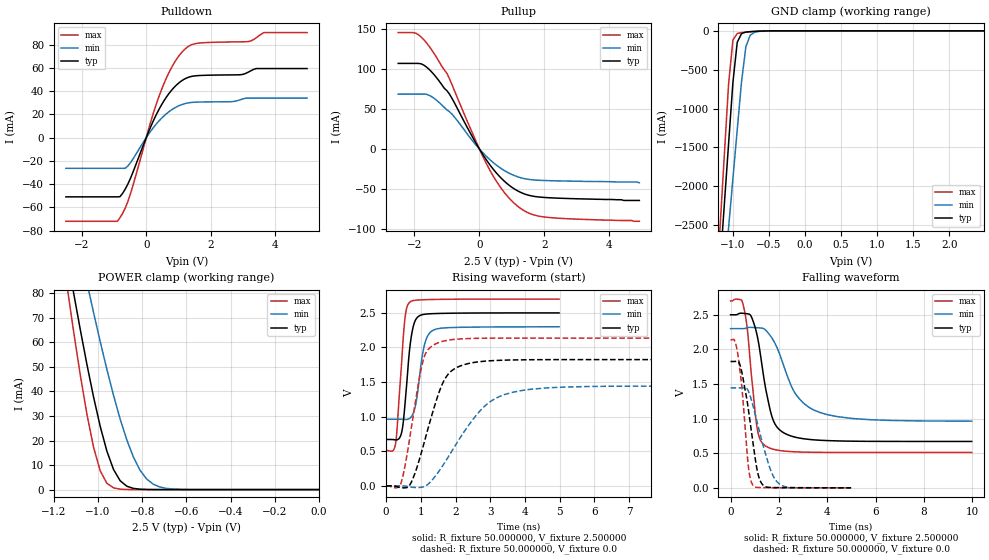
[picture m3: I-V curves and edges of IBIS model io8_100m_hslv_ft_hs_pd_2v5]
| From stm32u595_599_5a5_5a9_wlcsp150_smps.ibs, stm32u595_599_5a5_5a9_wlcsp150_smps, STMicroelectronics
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|   Model io8_100m_hslv_ft_hs_pd_2v5
[Model]  io8_100m_hslv_ft_hs_pd_2v5
Model_type I/O
Polarity   Non-Inverting
Enable   Active-Low
Vinl =   0.750000V
Vinh =   1.750000V
Vmeas =  1.250000V
Cref =   50.000000pF
Rref =   100.000000M
Vref =   0.0V
C_comp   3.340900pF   3.338500pF   3.380300pF
[Temperature Range]   25.000000   0.140000k   -40.000000
[Pullup Reference]   2.500000V   2.300000V   2.700000V
[Pulldown Reference]   0.0V   0.0V   0.0V
[POWER Clamp Reference]   2.500000V   2.300000V   2.700000V
[GND Clamp Reference]   0.0V   0.0V   0.0V
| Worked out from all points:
|   slope of the pulldown table from 0 to 0.375 V, typ, clamps not added: 16.1 ohm
|   slope of the pullup table from 0 to 0.375 V, typ, clamps not added: 16.6 ohm
|   GND clamp passes 1 mA (typ) near -0.50 V on its own axis
|   POWER clamp passes 1 mA (typ) near -0.86 V on its own axis
|   rising waveform, R_fixture 50.000000, V_fixture 2.500000: 20-80 % time 200ps typ, 230ps min, 180ps max; typ from 0.67 V to 2.5 V
|   rising waveform, R_fixture 50.000000, V_fixture 0.0: 20-80 % time 660ps typ, 1.22ns min, 424ps max; typ from 0 V to 1.82 V
|   falling waveform, R_fixture 50.000000, V_fixture 2.500000: 20-80 % time 568ps typ, 1.09ns min, 361ps max; typ from 2.5 V to 0.67 V
|   falling waveform, R_fixture 50.000000, V_fixture 0.0: 20-80 % time 467ps typ, 672ps min, 321ps max; typ from 1.82 V to 0 V
[Pulldown]
|Voltage   I(typ)   I(min)   I(max)
-2.5V     -51.01mA   -26.45mA   -72.04mA
-900mV    -51.01mA   -26.45mA   -72.04mA
-820mV    -50.89mA   -26.45mA   -69.09mA
-500mV    -35.59mA   -21.93mA   -49.09mA
140mV     9.489mA    5.639mA    13.76mA
460mV     27.5mA     16.25mA    40.22mA
860mV     43.07mA    25.18mA    63.88mA
1.26V     51.38mA    29.65mA    77.49mA
1.66V     53.45mA    30.63mA    81.42mA
3.18V     56.44mA    34.01mA    82.68mA
3.66V     59.44mA    34.01mA    90.42mA
5V        59.44mA    34.01mA    90.42mA
[Pullup]
|Voltage   I(typ)   I(min)   I(max)
-2.5V     106.7mA    68.56mA    145.2mA
-1.96V    106.7mA    68.56mA    144.4mA
-1.72V    104.8mA    68.56mA    136.6mA
-1.48V    96.52mA    65.55mA    124.2mA
-1V       72.68mA    48.88mA    94.22mA
-120mV    8.307mA    5.657mA    10.97mA
280mV     -17.4mA    -11.68mA   -23.32mA
680mV     -36.72mA   -24.56mA   -49.54mA
1.16V     -51.75mA   -34.32mA   -70.71mA
1.56V     -58mA      -38.01mA   -80.45mA
1.96V     -60.18mA   -39.11mA   -84.44mA
4.92V     -64mA      -42mA      -90mA
[GND_clamp]
|Voltage   I(typ)   I(min)   I(max)
-2.5V     -9.446A    -9.524A    -9.146A
-1.18V    -3.045A    -3.8A      -2.552A
-1.12V    -2.248A    -3.166A    -1.614A
-1.06V    -1.452A    -2.533A    -685.4mA
-1V       -665mA     -1.901A    -117.9mA
-940mV    -148mA     -1.272A    -34.34mA
-880mV    -35.14mA   -651.5mA   -22.8mA
-820mV    -16.02mA   -203.9mA   -17.08mA
-760mV    -10.47mA   -56.89mA   -12.28mA
-700mV    -7.079mA   -18.53mA   -8.16mA
-400mV    -112.4uA   -382.5uA   -53.84uA
2.48V     63.1uA     48.03uA    77.39uA
[POWER_clamp]
|Voltage   I(typ)   I(min)   I(max)
-2.49V    881mA      773.1mA    1.07A
-1.14V    95.25mA    122.7mA    82.82mA
-1.11V    79.9mA     109.7mA    64.14mA
-1.05V    50.87mA    84.26mA    30.57mA
-1.02V    37.63mA    72.04mA    17.17mA
-990mV    25.71mA    60.25mA    7.621mA
-930mV    8.217mA    38.43mA    713.9uA
-900mV    3.624mA    28.77mA    182.8uA
-840mV    490.7uA    13.24mA    11.35uA
-780mV    56.55uA    4.324mA    699nA
-660mV    716.5nA    226uA      9.775nA
0V        0A         19.49nA    0A
[Ramp]
| variable   typ   min   max
dV/dt_r  1.09464/0.65907n   0.86544/1.21762n   1.28142/0.42296n
dV/dt_f  1.09786/0.56759n   0.80138/1.08495n   1.31323/0.36111n
R_load = 50.000000
[Rising Waveform]
R_fixture= 50.000000
V_fixture= 2.500000
V_fixture_min= 2.300000
V_fixture_max= 2.700000
|time   V(typ)   V(min)   V(max)
0s        669.6mV    962.6mV    510.3mV
270.3ps   664.1mV    962.9mV    606.1mV
310.3ps   664.7mV    962.9mV    793.2mV
450.5ps   779.9mV    962.3mV    1.814V
550.6ps   1.223V     959.4mV    2.454V
680.7ps   1.991V     975.8mV    2.655V
860.9ps   2.409V     1.2V       2.683V
1.071ns   2.477V     1.964V     2.689V
1.301ns   2.487V     2.233V     2.693V
4.985ns   2.499V     2.299V     2.698V
[Rising Waveform]
R_fixture= 50.000000
V_fixture= 0.0
V_fixture_min= 0.0
V_fixture_max= 0.0
|time   V(typ)   V(min)   V(max)
0s        -146.1uV   -65.63uV   -358.7uV
400.4ps   -24.12mV   -179.5uV   3.553mV
680.7ps   11.58mV    -15.31mV   692.2mV
1.081ns   598mV      -13.76mV   1.838V
1.481ns   1.289V     181.9mV    2.065V
1.702ns   1.551V     346.1mV    2.097V
1.982ns   1.695V     573.8mV    2.117V
2.723ns   1.796V     1.092V     2.132V
3.423ns   1.816V     1.321V     2.135V
9.97ns    1.825V     1.442V     2.135V
[Falling Waveform]
R_fixture= 50.000000
V_fixture= 2.500000
V_fixture_min= 2.300000
V_fixture_max= 2.700000
|time   V(typ)   V(min)   V(max)
0s        2.499V     2.299V     2.698V
520.5ps   2.52V      2.298V     2.646V
700.7ps   2.513V     2.313V     2.269V
1.101ns   2.198V     2.312V     860.5mV
1.461ns   1.415V     2.274V     601.8mV
1.722ns   1.017V     2.157V     561.7mV
1.982ns   853mV      1.973V     541.5mV
2.623ns   736mV      1.393V     520.9mV
3.443ns   693mV      1.123V     513.2mV
9.97ns    669.6mV    962.6mV    510.3mV
[Falling Waveform]
R_fixture= 50.000000
V_fixture= 0.0
V_fixture_min= 0.0
V_fixture_max= 0.0
|time   V(typ)   V(min)   V(max)
0s        1.825V     1.442V     2.135V
160.2ps   1.825V     1.443V     2.131V
300.3ps   1.83V      1.443V     1.93V
470.5ps   1.665V     1.444V     1.442V
740.7ps   1.122V     1.394V     299.1mV
930.9ps   643.2mV    1.182V     35.74mV
1.271ns   72.54mV    711.4mV    3.759mV
1.662ns   5.383mV    250.7mV    1.862mV
2.002ns   2.943mV    60.39mV    982.9uV
4.985ns   -146.1uV   -65.63uV   -358.7uV
